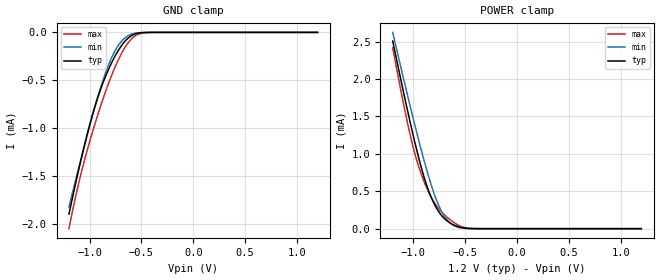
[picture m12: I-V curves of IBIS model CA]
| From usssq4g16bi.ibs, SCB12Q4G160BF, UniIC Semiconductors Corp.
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|   Model CA
[Model] CA
Model_type Input
Polarity   Non-Inverting
Enable   Active-High
Vinl =  5.100E-01
Vinh =  6.900E-01
C_comp   3.635E-13   3.578E-13   3.695E-13
C_comp_power_clamp   9.797E-14   9.219E-14   1.041E-13
C_comp_gnd_clamp   2.655E-13   2.655E-13   2.656E-13
[Model Spec]
Vinh   6.900E-01   6.600E-01   7.200E-01
Vinl   5.100E-01   4.800E-01   5.400E-01
[Temperature Range]   45.000   95.000   -40.000
[Voltage Range]   1.200E+00   1.140E+00   1.260E+00
[C Comp Corner]
C_comp_power_clamp   9.797E-14   1.041E-13   9.219E-14
C_comp_gnd_clamp   2.655E-13   2.655E-13   2.656E-13
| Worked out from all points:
|   GND clamp passes 1 mA (typ) near -1.01 V on its own axis
|   POWER clamp passes 1 mA (typ) near -0.96 V on its own axis
[GND_clamp]
|Voltage   I(typ)   I(min)   I(max)
-1.2V     -1.894mA   -1.82mA    -2.046mA
-1.125V   -1.523mA   -1.494mA   -1.661mA
-1.075V   -1.288mA   -1.282mA   -1.437mA
-975mV    -866.8uA   -874.7uA   -1.046mA
-900mV    -609.6uA   -596uA     -786.6uA
-825mV    -402.8uA   -357.9uA   -551.9uA
-750mV    -236.9uA   -181.2uA   -348.1uA
-675mV    -112.4uA   -72.29uA   -184.6uA
-575mV    -22.31uA   -11.6uA    -46.87uA
-500mV    -3.511uA   -1.89uA    -8.391uA
-425mV    -376nA     -250.4nA   -804.6nA
1.2V      0A         0A         0A
[POWER_clamp]
|Voltage   I(typ)   I(min)   I(max)
-1.2V     2.508mA    2.622mA    2.419mA
-1.125V   2.013mA    2.178mA    1.873mA
-1.05V    1.535mA    1.743mA    1.369mA
-1V       1.233mA    1.461mA    1.075mA
-950mV    950.9uA    1.187mA    832.5uA
-875mV    590.6uA    800.9uA    554.5uA
-800mV    333.4uA    466.5uA    350.8uA
-725mV    169.8uA    220.5uA    218.7uA
-650mV    79.35uA    80.24uA    123.5uA
-550mV    18.67uA    13.19uA    35.89uA
-425mV    849.8nA    680.9nA    1.522uA
1.2V      0A         0A         0A
